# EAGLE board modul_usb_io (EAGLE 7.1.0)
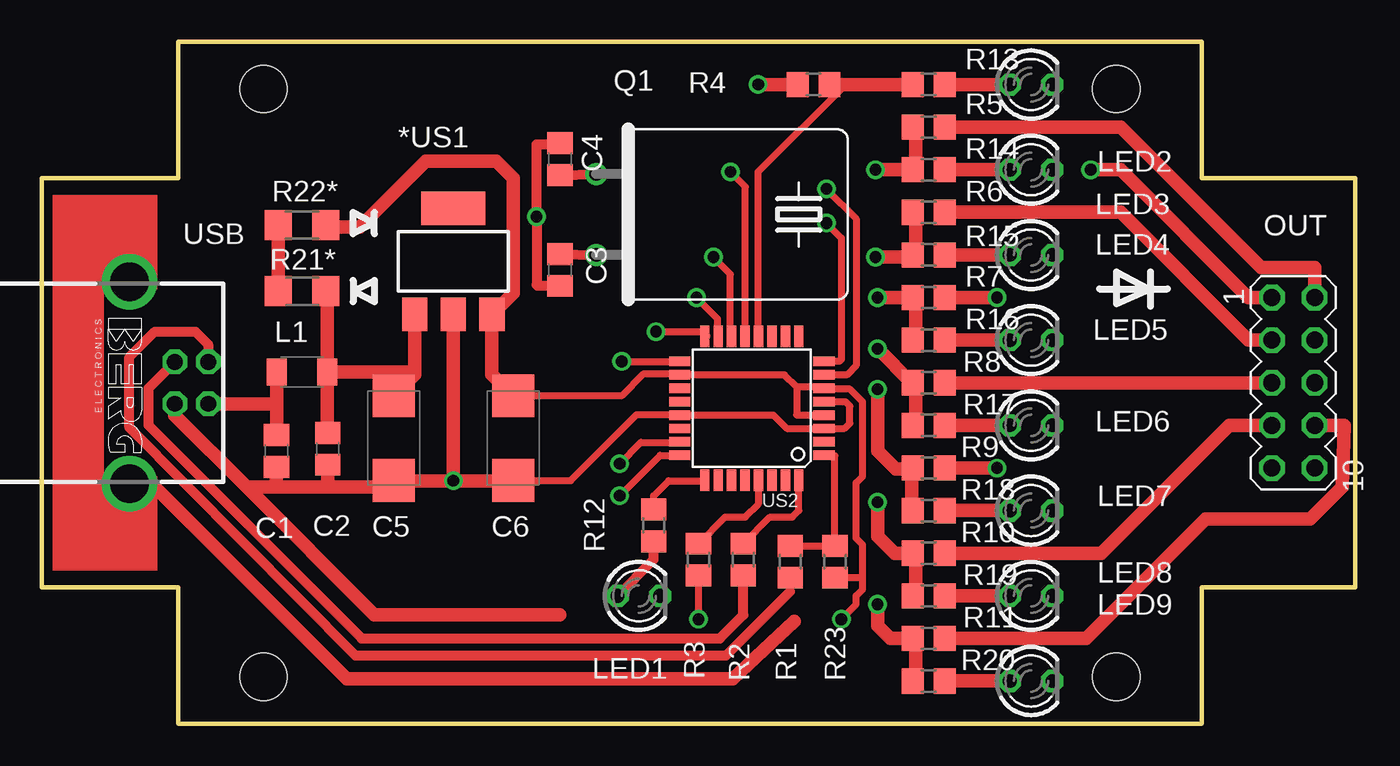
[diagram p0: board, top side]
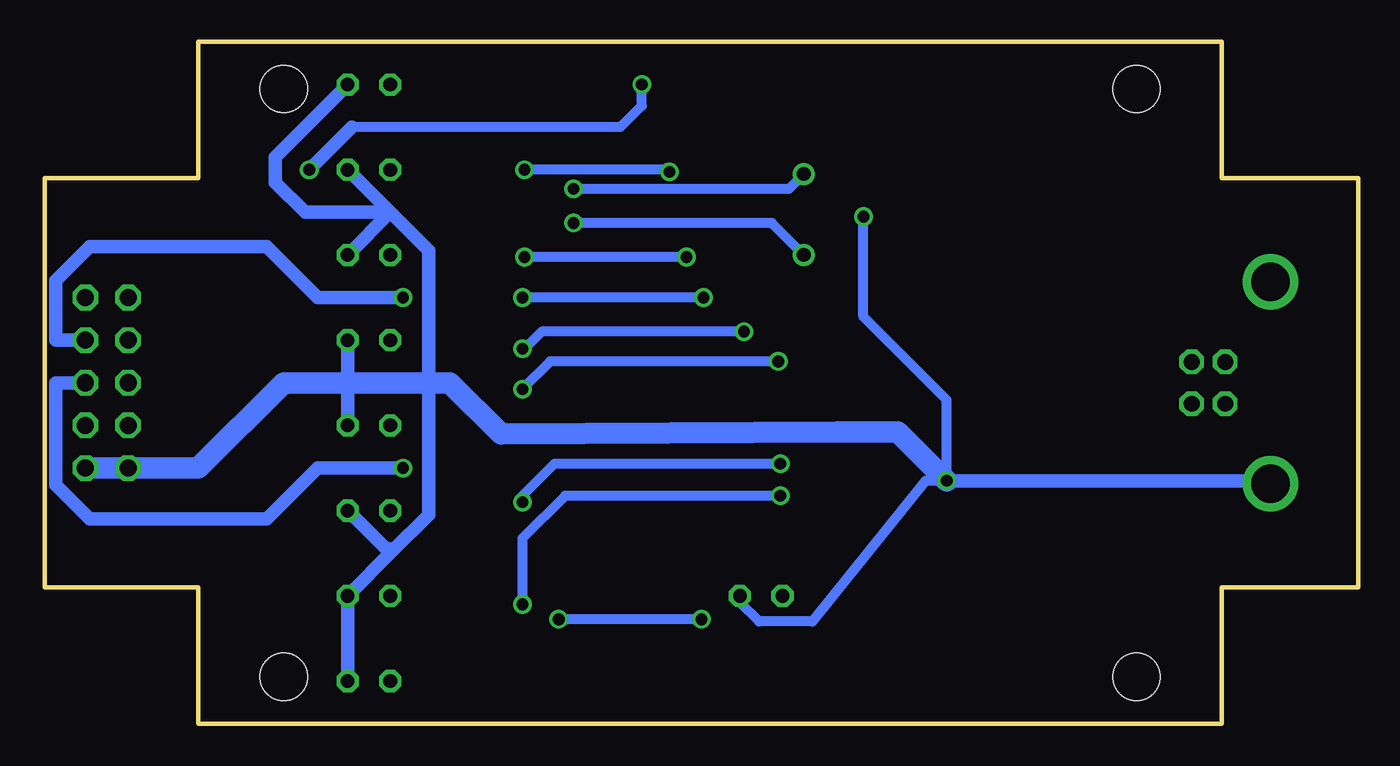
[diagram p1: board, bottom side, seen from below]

Size 78.23 x 40.64 mm. Coordinates in mm from the lower left corner, seen from the top.
Outline: 8.13,0 69.09,0 69.09,8.13 78.23,8.13 78.23,32.51 69.09,32.51 69.09,40.64 8.13,40.64 8.13,32.51 0,32.51 0,8.13 8.13,8.13 8.13,0
Copper layers (1*16): Top 0.035mm / dielectric 1.5mm / Bottom 0.035mm
Design rules "default": minimum track width 10mil, minimum drill 24mil, track to track 8mil, track to pad 8mil, pad to pad 8mil, via to via 8mil, smd to smd 8mil, copper to edge 40mil, drill to drill 8mil, minimum pad ring 10mil, minimum via ring 8mil, stop-mask expansion 4mil, vias tented up to drill 0mil, thermal gap 10mil
Holes 2.8 mm at 13.21,37.85 64.01,37.85 64.01,2.79 13.21,2.79

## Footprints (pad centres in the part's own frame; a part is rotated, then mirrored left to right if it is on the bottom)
SOT223 = smd 1.5 x 2: 1 -2.3,-3.15; 2 0,-3.15; 3 2.3,-3.15 | smd 3.8 x 2: 4 0,3.15
C0805 = smd 1.3 x 1.5: 1 -0.95,0; 2 0.95,0
C/6032-28R = smd 2.55 x 2.5: + 2.525,0; - -2.525,0
L3216C = smd 1.2 x 1.6: 1 -1.5,0; 2 1.5,0
LED3MM = drill 0.813 octagon: A -1.27,0; K 1.27,0
MA05-2 = drill 1.016 octagon: 1 -5.08,-1.27; 2 -5.08,1.27; 3 -2.54,-1.27; 4 -2.54,1.27; 5 0,-1.27; 6 0,1.27; 7 2.54,-1.27; 8 2.54,1.27; 9 5.08,-1.27; 10 5.08,1.27
HC49U-H = drill 0.813: 1 -2.413,-5.08; 2 2.413,-5.08
R0805 = smd 1.3 x 1.5: 1 -0.95,0; 2 0.95,0
R1206 = smd 1.6 x 1.803: 1 -1.422,0; 2 1.422,0
TQFP32-08 = smd 1.27 x 0.559: 1 -4.293,2.8; 2 -4.293,2; 3 -4.293,1.2; 4 -4.293,0.4; 5 -4.293,-0.4; 6 -4.293,-1.2; 7 -4.293,-2; 8 -4.293,-2.8; 17 4.293,-2.8; 18 4.293,-2; 19 4.293,-1.2; 20 4.293,-0.4; 21 4.293,0.4; 22 4.293,1.2; 23 4.293,2; 24 4.293,2.8 | smd 0.559 x 1.27: 9 -2.8,-4.293; 10 -2,-4.293; 11 -1.2,-4.293; 12 -0.4,-4.293; 13 0.4,-4.293; 14 1.2,-4.293; 15 2,-4.293; 16 2.8,-4.293; 25 2.8,4.293; 26 2,4.293; 27 1.2,4.293; 28 0.4,4.293; 29 -0.4,4.293; 30 -1.2,4.293; 31 -2,4.293; 32 -2.8,4.293
PN61729-S = drill 0.95 octagon: 1 1.25,4.71; 2 -1.25,4.71; 3 -1.25,2.71; 4 1.25,2.71 | drill 2.3 pad 2.9: S1 -6.02,0; S2 6.02,0

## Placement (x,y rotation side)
*US1  [SOT223]  24.51,27.56 0 top
C1  100nF  [C0805]  13.97,16.26 270 top
C2  100nF  [C0805]  17.02,16.38 270 top
C3  18pF  [C0805]  30.86,27.05 90 top
C4  18pF  [C0805]  30.86,33.66 90 top
C5  10uF  [C/6032-28R]  20.95,17.02 90 top
C6  10uF  [C/6032-28R]  28.07,17.02 90 top
L1  10uH  [L3216C]  15.49,20.95 0 top
LED1  [LED3MM]  35.56,7.62 0 top
LED2  [LED3MM]  58.93,38.1 0 top
LED3  [LED3MM]  58.93,33.02 0 top
LED4  [LED3MM]  58.93,27.94 0 top
LED5  [LED3MM]  58.93,22.86 0 top
LED6  [LED3MM]  58.93,17.78 0 top
LED7  [LED3MM]  58.93,12.7 0 top
LED8  [LED3MM]  58.93,7.62 0 top
LED9  [LED3MM]  58.93,2.54 0 top
OUT  [MA05-2]  74.55,20.32 270 top
Q1  12MHz  [HC49U-H]  38.1,30.35 270 top
R1  22R  [R0805]  44.58,9.65 90 top
R2  22R  [R0805]  41.78,9.78 90 top
R3  3.3k  [R0805]  39.12,9.78 90 top
R4  [R0805]  45.97,38.1 180 top
R5  [R0805]  52.83,35.56 0 top
R6  [R0805]  52.83,30.48 0 top
R7  [R0805]  52.83,25.4 0 top
R8  [R0805]  52.83,20.32 0 top
R9  [R0805]  52.83,15.24 0 top
R10  [R0805]  52.83,10.16 0 top
R11  [R0805]  52.83,5.08 0 top
R12  [R0805]  36.45,11.81 270 top
R13  [R0805]  52.83,38.1 0 top
R14  [R0805]  52.83,33.02 0 top
R15  [R0805]  52.83,27.94 0 top
R16  [R0805]  52.83,22.86 0 top
R17  [R0805]  52.83,17.78 0 top
R18  [R0805]  52.83,12.7 0 top
R19  [R0805]  52.83,7.62 0 top
R20  [R0805]  52.83,2.54 0 top
R21*  [R1206]  15.49,25.78 180 top
R22*  [R1206]  15.49,29.72 0 top
R23  1.5k  [R0805]  47.24,9.65 270 top
US2  MEGA8  [TQFP32-08]  42.29,18.8 180 top
USB  [PN61729-S]  5.21,20.32 270 top

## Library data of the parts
*US1 = v-reg
C1-C6 L1 R1-R20 R21* R22* R23 = rcl
LED1-LED9 = led
OUT = con-lstb
Q1 = crystal
US2 = avr-4
USB = con-berg

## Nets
GND: *US1.2 C1.2 C2.2 C3.1 C4.2 C5.- C6.- LED1.K LED2.K LED3.K LED4.K LED5.K LED6.K LED7.K LED8.K LED9.K OUT.9 OUT.10 US2.3 US2.5 US2.21 USB.4 USB.S1 USB.S2
IO1: R4.1 R13.1 US2.12
IO2: R5.1 R14.1 US2.13
IO3: R6.1 R15.1 US2.14
IO4: R7.1 R16.1 US2.15
IO5: R8.1 R17.1 US2.16
IO6: R9.1 R18.1 US2.17
IO7: R10.1 R19.1 US2.23
IO8: R11.1 R20.1 US2.24
LED: R12.1 US2.25
N$1: *US1.1 C2.1 C5.+ L1.2 R21*.1
N$2: R21*.2 R22*.1
N$3: C4.1 Q1.1 US2.7
N$4: C3.2 Q1.2 US2.8
N$5: C1.1 L1.1 USB.1
N$6: OUT.4 R7.2
N$8: R3.2 US2.29
N$9: R1.1 USB.2
N$10: R2.1 USB.3
N$24: LED2.A R13.2
N$25: LED3.A R14.2
N$26: LED4.A R15.2
N$27: LED5.A R16.2
N$28: LED6.A R17.2
N$29: LED7.A R18.2
N$30: LED8.A R19.2
N$31: LED9.A R20.2
N$32: LED1.A R12.2
N$35: OUT.8 R11.2
N$36: OUT.6 R9.2
N$37: OUT.2 R5.2
N$38: OUT.1 R4.2
N$39: OUT.3 R6.2
N$40: OUT.5 R8.2
N$41: OUT.7 R10.2
USBA: R2.2 US2.32
USBB: R1.2 R23.1 US2.1
V+: *US1.3 C6.+ R3.1 R22*.2 R23.2 US2.4 US2.6 US2.18

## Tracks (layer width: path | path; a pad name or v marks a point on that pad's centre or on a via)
GND  (via drill 0.7 pad 1.02)
  Top 0.406: US2.5 46.6,19.18 47.88,19.18 48.13,18.92 48.13,17.91 47.82,17.6 US2.3 44.38,17.6 43.58,18.4 US2.21 38.02,18.41 35.43,18.41 31.51,14.49 C6.-
  Top 0.61: C4.2 30.8,34.54 29.46,34.54 v29.46,30.23 29.46,26.16 29.53,26.1 C3.1
  Top 0.813: v24.51,14.48 28.05,14.48 C6.- | 13.97,14.1 C1.2 | 17.14,14.1 13.97,14.1 | 17.14,14.1 20.56,14.1 C5.- 20.97,14.48 v24.51,14.48 | C2.2 17.02,14.22 17.14,14.1 | USB.4 7.92,18.37 12.19,14.1 | 13.97,14.1 12.19,14.1 | 12.19,14.1 19.81,6.48 30.86,6.48 | v24.51,14.48 *US1.2 | USB.S1 5.16,26.29 3.3,26.29 3.17,26.16 3.17,14.35 3.23,14.3 USB.S2
  Bottom 0.61: LED1.K 36.83,7.24 35.69,6.1 32.51,6.1 25.78,14.48 v24.51,14.48 24.51,19.3 29.46,24.26 v29.46,30.23
  Bottom 0.813: 57.66,30.48 55.37,28.19 55.37,20.32 55.37,12.45 57.53,10.29 | 57.66,30.48 LED3.K | 57.66,30.48 LED4.K | LED5.K 60.2,20.32 LED6.K | 57.53,10.29 LED8.K LED9.K | 57.53,10.29 57.66,10.41 57.91,10.41 LED7.K | LED2.K 64.52,33.78 64.52,32.26 62.74,30.48 57.66,30.48 | USB.S2 5.38,14.48 v24.51,14.48
  Bottom 1.27: OUT.10 OUT.9 69.09,15.24 64.01,20.32 60.2,20.32 55.37,20.32 54.1,20.32 51.05,17.27 30.99,17.4 27.43,17.4 v24.51,14.48
IO1
  Top 0.406: US2.12 42.67,23.11 42.67,32.89 47.88,38.1 | 49.02,38.1 48.89,38.1
  Top 0.813: 52.07,38.1 R13.1 49.02,38.1 47.88,38.1 R4.1
IO2  (via drill 0.7 pad 1.02)
  Top 0.406: US2.13 41.91,23.2 41.91,32 v41.02,32.89
  Top 0.813: 51.94,33.02 52.07,33.02 52.07,35.37 R5.1 | 51.94,33.02 R14.1 | v49.66,33.02 51.94,33.02
  Bottom 0.61: 41.15,33.02 v49.66,33.02
  Bottom 0.813: v41.02,32.89 41.15,33.02
IO3  (via drill 0.7 pad 1.02)
  Top 0.406: US2.14 41.02,23.16 41.02,26.8 v40,27.81
  Top 0.813: R6.1 52.07,30.29 52.07,28.13 R15.1 51.75,27.81 v49.66,27.81
  Bottom 0.61: v40,27.81 v49.66,27.81
IO4  (via drill 0.7 pad 1.02)
  Top 0.406: US2.15 40.27,23.11 40.26,23.11 40.26,24.13 v38.99,25.4
  Top 0.813: R16.1 52.07,23.05 52.07,25.02 51.69,25.4 | R7.1 52.07,25.21 | v49.78,25.4 R7.1 | 51.69,25.4 51.56,25.53 | R7.1 51.69,25.4
  Bottom 0.61: v38.99,25.4 v49.78,25.4
IO5  (via drill 0.7 pad 1.02)
  Top 0.406: US2.16 39.6,23.09 39.62,23.11 39.37,23.37 v36.58,23.37
  Top 0.813: R17.1 52.07,17.78 52.07,20.13 R8.1 51.82,20.32 v49.78,22.35
  Bottom 0.61: 49.66,22.35 48.64,23.37 v36.58,23.37
  Bottom 0.813: 49.66,22.35 v49.78,22.35
IO6  (via drill 0.7 pad 1.02)
  Top 0.406: US2.17 v34.54,21.59
  Top 0.813: 51.82,12.63 51.82,12.45 | 51.82,12.63 R18.1 | 51.82,15.17 R9.1 | 51.82,15.17 51.82,12.63 | 51.82,15.17 50.87,15.17 49.78,16.26 v49.78,19.94
  Bottom 0.61: v49.78,19.94 48.13,21.59 v34.54,21.59
IO7  (via drill 0.7 pad 1.02)
  Top 0.406: US2.23 38.1,16.89 | US2.23 | v34.42,15.49 35.69,16.76 37.97,16.76 US2.23
  Top 0.813: R19.1 52.07,7.62 52.07,9.97 R10.1 50.8,10.16 49.78,11.18 v49.78,13.21
  Bottom 0.61: v49.78,13.21 49.78,13.59 47.88,15.49 v34.42,15.49
IO8  (via drill 0.7 pad 1.02)
  Top 0.406: US2.24 36.82,16 v34.42,13.59
  Top 0.813: R20.1 52.07,2.54 52.07,4.89 R11.1 | v49.78,7.11 49.78,5.84 50.55,5.08 R11.1 | R11.1 52.07,5.08
  Bottom 0.61: v34.42,13.59 47.24,13.59 49.78,11.05 v49.78,7.11
LED
  Top 0.406: R12.1 36.45,13.59 37.34,14.48 39.47,14.48 US2.25
N$1
  Top 0.813: *US1.1 22.21,20.8 22.11,20.69 | 22.11,20.69 C5.+ | L1.2 16.99,17.36 C2.1 | L1.2 21.84,20.95 22.11,20.69 | L1.2 16.99,25.7 R21*.1
N$2
  Top 0.813: R21*.2 R22*.1
N$3  (via drill 0.7 pad 1.02)
  Top 0.406: US2.7 47.97,20.8 48.51,21.34 48.51,30.1 v46.74,31.88
  Top 0.61: C4.1 Q1.1
  Bottom 0.61: v46.74,31.88 33.91,31.88 Q1.1
N$4  (via drill 0.7 pad 1.02)
  Top 0.406: US2.8 47.5,21.6 47.62,21.72 47.62,28.96 v46.74,29.84
  Top 0.61: C3.2 Q1.2
  Bottom 0.61: v46.74,29.84 34.92,29.84 Q1.2
N$5
  Top 0.813: 13.99,19.18 13.99,17.23 C1.1 | 13.99,19.18 L1.1 | USB.1 13.89,19.07 13.99,19.18
N$6  (via drill 0.7 pad 1.02)
  Top 0.813: R7.2 v56.9,25.4
  Bottom 0.813: OUT.4 77.6,22.86 77.6,26.42 75.56,28.45 65.02,28.45 61.98,25.4 v56.9,25.4
N$7
  Top 0.813: 6.6,14.22 18.16,2.67 41.15,2.67 44.83,6.1
N$8
  Top 0.406: US2.29 42.69,13.1 41.91,12.32 40.71,12.32 R3.2
N$9
  Top 0.406: 44.58,7.87 R1.1 | 9.91,21.58 USB.2
  Top 0.61: 44.58,7.87 40.77,4.06 18.67,4.06 5.21,17.65 5.21,21.84 6.73,23.37 9.14,23.37 9.91,22.61 9.91,21.58
N$10
  Top 0.61: R2.1 41.78,6.48 40.39,5.08 19.05,5.08 6.35,17.78 6.35,20 USB.3
N$24
  Top 0.813: R13.2 LED2.A
N$25
  Top 0.813: R14.2 LED3.A
N$26
  Top 0.813: R15.2 LED4.A
N$27
  Top 0.813: R16.2 LED5.A
N$28
  Top 0.813: R17.2 LED6.A
N$29
  Top 0.813: R18.2 LED7.A
N$30
  Top 0.813: R19.2 LED8.A
N$31
  Top 0.813: R20.2 LED9.A
N$32
  Top 0.61: R12.2 36.45,9.78 LED1.A
N$35
  Top 0.813: OUT.8 77.6,17.78 77.47,14.1 75.56,12.19 69.34,12.19 62.23,5.08 R11.2 53.59,5.08
N$36  (via drill 0.7 pad 1.02)
  Top 0.813: 53.59,15.24 R9.2 v56.9,15.24
  Bottom 0.813: OUT.6 77.6,20.32 77.6,14.22 75.56,12.19 65.02,12.19 61.98,15.24 v56.9,15.24
N$37
  Top 0.813: OUT.2 75.82,27.18 72.64,27.18 64.26,35.56 R5.2
N$38  (via drill 0.7 pad 1.02)
  Top 0.813: OUT.1 71.88,25.4 64.26,33.02 v62.48,33.02 | v42.67,38.1 R4.2
  Bottom 0.61: 59.94,35.56 43.94,35.56 42.67,36.83 v42.67,38.1
  Bottom 0.813: 59.94,35.56 v62.48,33.02
N$39
  Top 0.813: OUT.3 71.88,22.86 64.26,30.48 R6.2
N$40
  Top 0.813: R8.2 OUT.5
N$41
  Top 0.813: OUT.7 70.74,17.78 63.12,10.16 R10.2
USBA
  Top 0.406: US2.32 45.09,12.71 44.7,12.32 43.37,12.32 R2.2
USBB
  Top 0.406: US2.1 47.24,15.97 R23.1 R1.2
V+  (via drill 0.7 pad 1.02)
  Top 0.406: 44.96,20.07 44.23,20.8 US2.18 37.97,20.83 35.81,20.83 34.53,19.54 C6.+ | 44.96,20.07 46.51,20.07 US2.6 46.64,19.94 48.13,19.94 48.89,19.18 48.89,14.73 48.51,14.35 48.51,11.05 48.89,10.67 48.89,8.64 | US2.4 44.98,18.4 44.96,18.41 44.96,20.07 | 48.89,8.64 48.89,8 48.51,7.62 48.51,7.11 v47.62,6.22 | R23.2 48.83,8.7 48.89,8.64 | v39.12,6.22 R3.1
  Top 0.813: 26.81,24.4 26.81,20.8 C6.+ | 26.81,24.4 *US1.3 | 26.81,24.4 28.07,25.65 28.07,32.51 27.05,33.53 22.86,33.53 18.92,29.59 17.04,29.59 R22*.2
  Bottom 0.61: v39.12,6.22 v47.62,6.22
(copper drawn outside any net)
  shapes: Top area x3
